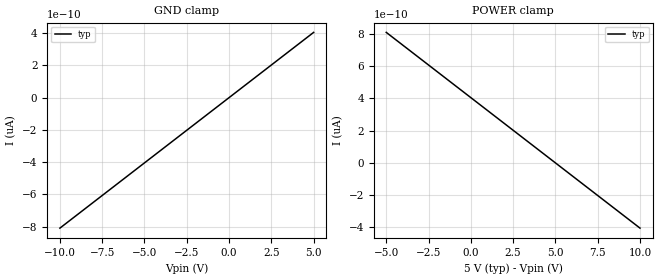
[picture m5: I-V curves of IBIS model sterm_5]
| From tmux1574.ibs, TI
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| sterm_5
[Model]   sterm_5
Model_type   Terminator
|   typ   min   max
C_comp   4.014581e-12   NA   NA
[Voltage Range]   5   NA   NA
[Temperature Range]   27   NA   NA
[Power Clamp Reference]   5   NA   NA
[GND Clamp Reference]   0   NA   NA
[GND Clamp]
|   Voltage   I(typ)   I(min)   I(max)
-10V      0A         NA         NA
454.5mV   0A         NA         NA
606.1mV   0A         NA         NA
5V        0A         NA         NA
[POWER Clamp]
|   Voltage   I(typ)   I(min)   I(max)
-5V       0A         NA         NA
-4.091V   0A         NA         NA
-3.939V   0A         NA         NA
10V       0A         NA         NA
